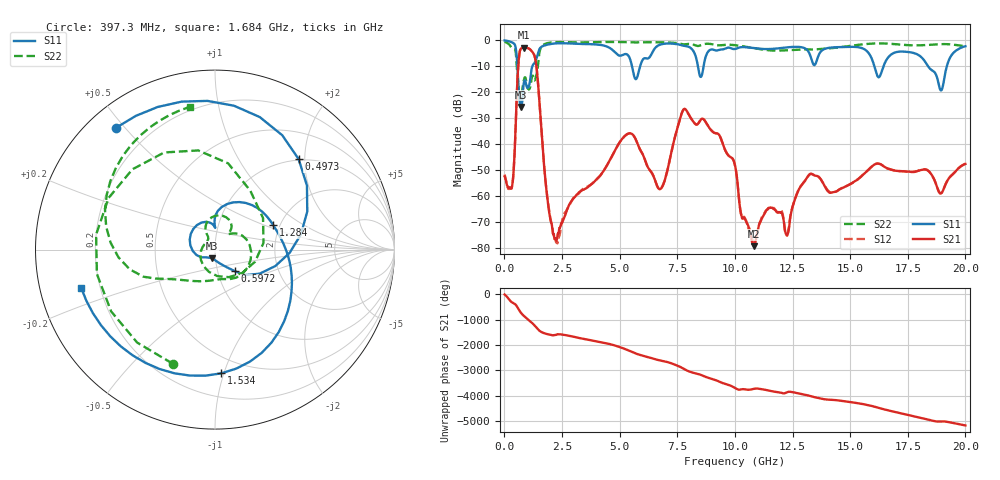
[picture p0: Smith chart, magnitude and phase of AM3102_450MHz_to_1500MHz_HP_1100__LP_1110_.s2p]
!Agilent Technologies,E8364B,MY43040894,A.07.50.67
!Agilent E8364B: A.07.50.67
!Date: Thursday, January 11, 2018 06:36:09
!Correction: S11(Full 2 Port(1,2))
!S21(Full 2 Port(1,2))
!S12(Full 2 Port(1,2))
!S22(Full 2 Port(1,2))
!S2P File: Measurements: S11, S21, S12, S22:
# Hz S  dB  R 50
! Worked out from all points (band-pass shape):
!   1601 points, 10 MHz to 20 GHz, reference 50 ohm
!   highest |S21| = -2.90 dB at 847.1 MHz (marker M1); lowest = -79.5 dB at 10.83 GHz (marker M2)
!   |S21| within 3 dB of the highest: 642.1 MHz to 1.301 GHz (659.2 MHz wide, 67.8 % of centre)
!   lowest |S11| = -25.8 dB at 722.1 MHz (marker M3), VSWR 1.11, Z = 47.9 - j4.58 ohm
!   |S11| at or under -10 dB: 565.5 MHz to 1.215 GHz (649.2 MHz wide, 72.9 % of centre); 16.05 GHz to 16.45 GHz (400 MHz wide, 2.46 % of centre); 18.38 GHz to 19.2 GHz (819.8 MHz wide, 4.36 % of centre)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
!   |S22| runs from -23.9 to -0.5 dB; largest |S21 - S12| = 0.00065
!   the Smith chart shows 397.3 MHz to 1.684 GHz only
!   S11 on the Smith chart (normalised r, x): 397.3 MHz: 0.08, +0.47; 497.3 MHz: 0.98, +1.87; 597.2 MHz: 1.21, -0.30; 1.284 GHz: 1.84, +0.58; 1.534 GHz: 0.37, -0.98; 1.684 GHz: 0.13, -0.14
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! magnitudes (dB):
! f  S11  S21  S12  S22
! 10 MHz  -0.1  -52.6  -51.8  -0.5
! 397.3 MHz  -1.2  -50.9  -50.9  -3.4
! 497.3 MHz  -3.3  -30.9  -31.0  -5.0
! 597.2 MHz  -15.7  -10.5  -10.5  -16.6
! 722.1 MHz  -25.8  -3.2  -3.2  -23.3
! 847.1 MHz  -16.4  -2.9  -2.9  -15.3
! 1.284 GHz  -9.1  -5.5  -5.5  -15.2
! 1.534 GHz  -3.2  -25.8  -25.8  -4.2
! 1.684 GHz  -2.2  -44.1  -44.1  -1.9
! 2.221 GHz  -1.2  -76.4  -77.1  -0.7
! 3.346 GHz  -1.4  -58.1  -57.9  -0.9
! 5.432 GHz  -6.8  -35.9  -35.9  -0.8
! 6.682 GHz  -2.0  -57.1  -57.2  -0.8
! 7.819 GHz  -2.2  -26.5  -26.5  -1.6
! 10.01 GHz  -3.4  -48.3  -48.4  -1.9
! 10.83 GHz  -3.1  -79.5  -78.1  -3.1
! 11.53 GHz  -3.4  -64.6  -64.5  -3.9
! 12.25 GHz  -2.8  -75.4  -75.0  -3.9
! 13.34 GHz  -7.9  -51.6  -51.7  -3.6
! 16.68 GHz  -6.4  -49.6  -49.7  -1.3
! 18.94 GHz  -19.4  -59.1  -59.0  -1.5
! 20 GHz  -2.3  -47.8  -47.6  -2.3
